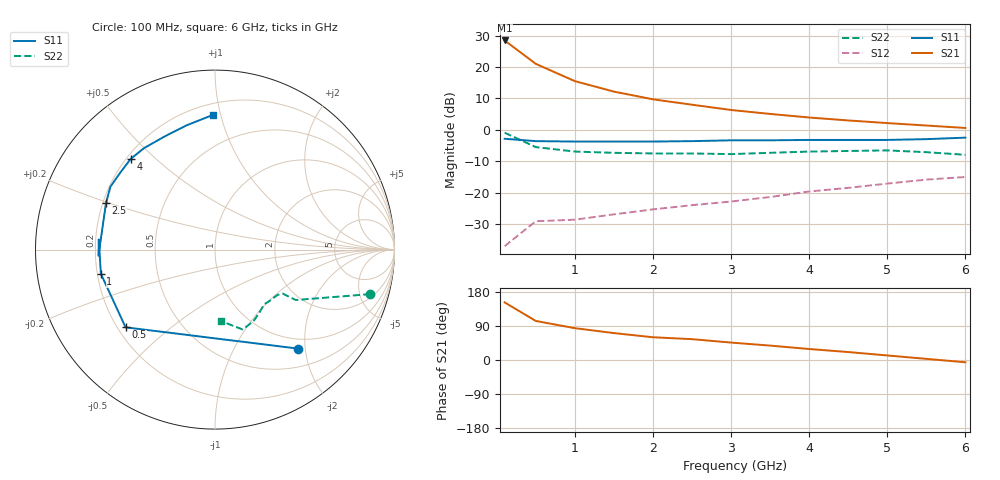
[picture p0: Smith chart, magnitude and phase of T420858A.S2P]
! AT-42085
!S AND NOISE PARAMETERS at Vce=8V  Ic=10mA.  LAST UPDATED 07-21-92
# ghz s ma r 50
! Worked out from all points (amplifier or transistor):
!   13 points, 100 MHz to 6 GHz, reference 50 ohm
!   highest |S21| = 28.5 dB at 100 MHz (marker M1)
!   |S21| within 3 dB of that: start of sweep to 260.8 MHz
!   unconditionally stable (mu >= 1): 1.215 GHz to 4.667 GHz
!   at 1 GHz: K = 0.92, MSG = 22.1 dB, |S12| = -28.6 dB
!   at 3 GHz: K = 1.30, MAG = 11.3 dB, |S12| = -22.9 dB
!   at 6 GHz: K = 0.83, MSG = 7.8 dB, |S12| = -15.0 dB
!   lowest NFmin = 1.10 dB at 100 MHz
!   S11 on the Smith chart (normalised r, x): 100 MHz: 0.81, -1.86; 500 MHz: 0.23, -0.36; 1 GHz: 0.21, -0.10; 2.5 GHz: 0.21, +0.19; 4 GHz: 0.22, +0.42; 6 GHz: 0.28, +0.94
0.1  0.72 -50.0  26.52 152.0  0.014 73.0  0.9 -16.0
0.5  0.66 -139.0  11.23 103.0  0.035 36.0  0.53 -32.0
1  0.65 -168.0  5.96 84.0  0.037 39.0  0.45 -33.0
1.5  0.65 175.0  4.06 71.0  0.045 46.0  0.43 -36.0
2  0.65 183.0  3.06 60.0  0.054 51.0  0.42 -41.0
2.5  0.66 157.0  2.51 55.0  0.063 60.0  0.42 -42.0
3  0.68 149.0  2.07 46.0  0.072 65.0  0.41 -48.0
3.5  0.68 141.0  1.79 38.0  0.085 64.0  0.43 -55.0
4  0.69 133.0  1.57 29.0  0.104 64.0  0.45 -61.0
4.5  0.69 125.0  1.41 21.0  0.119 63.0  0.46 -66.0
5  0.69 114.0  1.28 12.0  0.139 58.0  0.47 -71.0
5.5  0.71 103.0  1.17 3.0  0.161 55.0  0.44 -76.0
6  0.75 91.0  1.07 -6.0  0.177 49.0  0.4 -85.0
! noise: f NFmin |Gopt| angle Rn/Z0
0.1  1.1  0.05  16  0.13
0.5  1.2  0.06  77  0.13
1  1.3  0.1  131  0.12
2  2  0.24  -179  0.11
4  3.5  0.46  -128  0.25
